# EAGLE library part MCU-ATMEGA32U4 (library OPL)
8-bit Microcontroller with 16/32K Bytes of ISP Flash and USB Controller
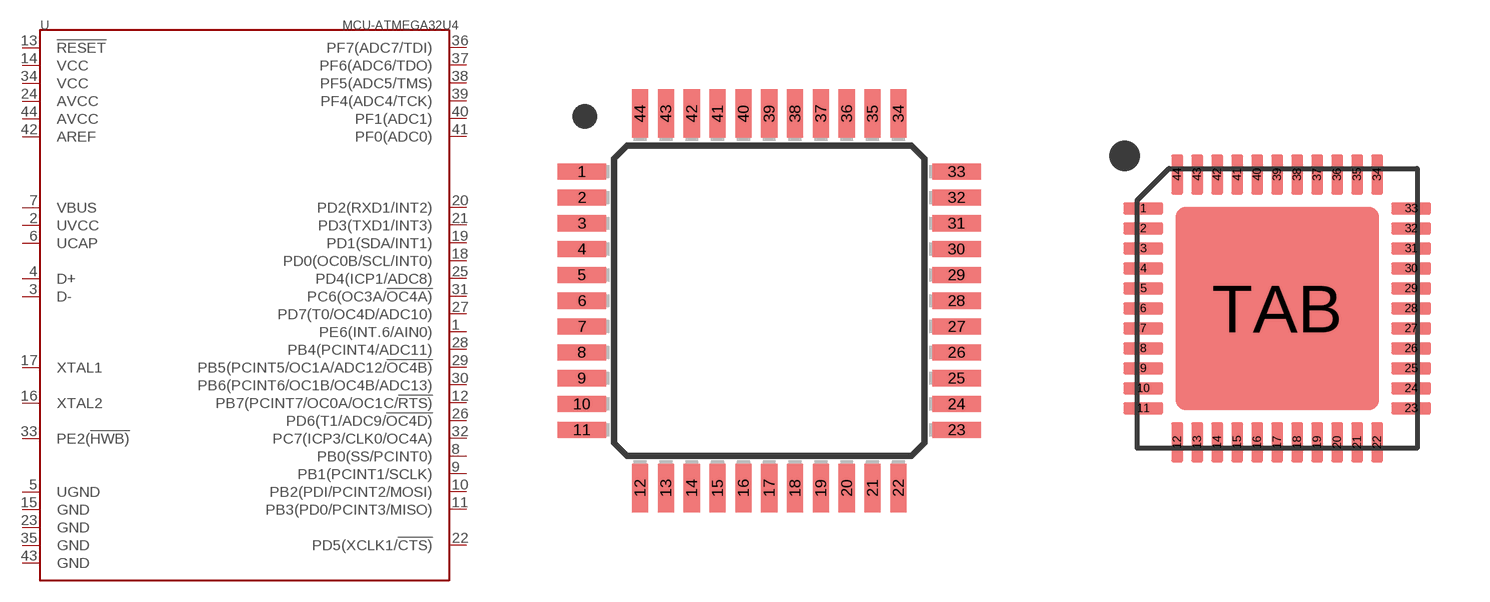
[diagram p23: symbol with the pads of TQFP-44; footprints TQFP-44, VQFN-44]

Designator prefix U

## MCU-ATMEGA32U4-310010010  [TQFP-44]
1  PE6(INT.6/AIN0)
2  UVCC
3  D-
4  D+
5  UGND
6  UCAP
7  VBUS
8  PB0(SS/PCINT0)
9  PB1(PCINT1/SCLK)
10  PB2(PDI/PCINT2/MOSI)
11  PB3(PD0/PCINT3/MISO)
12  PB7(PCINT7/OC0A/OC1C/!RTS)
13  !RESET
14  VCC
15  GND
16  XTAL2
17  XTAL1
18  PD0(OC0B/SCL/INT0)
19  PD1(SDA/INT1)
20  PD2(RXD1/INT2)
21  PD3(TXD1/INT3)
22  PD5(XCLK1/!CTS)
23  GND
24  AVCC
25  PD4(ICP1/ADC8)
26  PD6(T1/ADC9/!OC4D)
27  PD7(T0/OC4D/ADC10)
28  PB4(PCINT4/ADC11)
29  PB5(PCINT5/OC1A/ADC12/!OC4B)
30  PB6(PCINT6/OC1B/OC4B/ADC13)
31  PC6(OC3A/!OC4A)
32  PC7(ICP3/CLK0/OC4A)
33  PE2(!HWB)
34  VCC
35  GND
36  PF7(ADC7/TDI)
37  PF6(ADC6/TDO)
38  PF5(ADC5/TMS)
39  PF4(ADC4/TCK)
40  PF1(ADC1)
41  PF0(ADC0)
42  AREF
43  GND
44  AVCC

## MCU-ATMEGA32U4-310010016  [VQFN-44]
1  PE6(INT.6/AIN0)
2  UVCC
3  D-
4  D+
5  UGND
6  UCAP
7  VBUS
8  PB0(SS/PCINT0)
9  PB1(PCINT1/SCLK)
10  PB2(PDI/PCINT2/MOSI)
11  PB3(PD0/PCINT3/MISO)
12  PB7(PCINT7/OC0A/OC1C/!RTS)
13  !RESET
14  VCC
15  GND
16  XTAL2
17  XTAL1
18  PD0(OC0B/SCL/INT0)
19  PD1(SDA/INT1)
20  PD2(RXD1/INT2)
21  PD3(TXD1/INT3)
22  PD5(XCLK1/!CTS)
23  GND
24  AVCC
25  PD4(ICP1/ADC8)
26  PD6(T1/ADC9/!OC4D)
27  PD7(T0/OC4D/ADC10)
28  PB4(PCINT4/ADC11)
29  PB5(PCINT5/OC1A/ADC12/!OC4B)
30  PB6(PCINT6/OC1B/OC4B/ADC13)
31  PC6(OC3A/!OC4A)
32  PC7(ICP3/CLK0/OC4A)
33  PE2(!HWB)
34  VCC
35  GND
36  PF7(ADC7/TDI)
37  PF6(ADC6/TDO)
38  PF5(ADC5/TMS)
39  PF4(ADC4/TCK)
40  PF1(ADC1)
41  PF0(ADC0)
42  AREF
43  GND
44  AVCC
TAB  GND

## Footprint TQFP-44 (pad centres in mm)
Thin Plasic Quad Flat Package
smd 1.5 x 0.5: 1 -5.8,4; 2 -5.8,3.2; 3 -5.8,2.4; 4 -5.8,1.6; 5 -5.8,0.8; 6 -5.8,0; 7 -5.8,-0.8; 8 -5.8,-1.6; 9 -5.8,-2.4; 10 -5.8,-3.2; 11 -5.8,-4; 23 5.8,-4; 24 5.8,-3.2; 25 5.8,-2.4; 26 5.8,-1.6; 27 5.8,-0.8; 28 5.8,0; 29 5.8,0.8; 30 5.8,1.6; 31 5.8,2.4; 32 5.8,3.2; 33 5.8,4
smd 0.5 x 1.5: 12 -4,-5.8; 13 -3.2,-5.8; 14 -2.4,-5.8; 15 -1.6,-5.8; 16 -0.8,-5.8; 17 0,-5.8; 18 0.8,-5.8; 19 1.6,-5.8; 20 2.4,-5.8; 21 3.2,-5.8; 22 4,-5.8; 34 4,5.8; 35 3.2,5.8; 36 2.4,5.8; 37 1.6,5.8; 38 0.8,5.8; 39 0,5.8; 40 -0.8,5.8; 41 -1.6,5.8; 42 -2.4,5.8; 43 -3.2,5.8; 44 -4,5.8

## Footprint VQFN-44 (pad centres in mm)
smd 1 x 0.3: 1 -3.35,2.5; 2 -3.35,2; 3 -3.35,1.5; 4 -3.35,1; 5 -3.35,0.5; 6 -3.35,0; 7 -3.35,-0.5; 8 -3.35,-1; 9 -3.35,-1.5; 10 -3.35,-2; 11 -3.35,-2.5; 23 3.35,-2.5; 24 3.35,-2; 25 3.35,-1.5; 26 3.35,-1; 27 3.35,-0.5; 28 3.35,0; 29 3.35,0.5; 30 3.35,1; 31 3.35,1.5; 32 3.35,2; 33 3.35,2.5
smd 0.3 x 1: 12 -2.5,-3.35; 13 -2,-3.35; 14 -1.5,-3.35; 15 -1,-3.35; 16 -0.5,-3.35; 17 0,-3.35; 18 0.5,-3.35; 19 1,-3.35; 20 1.5,-3.35; 21 2,-3.35; 22 2.5,-3.35; 34 2.5,3.35; 35 2,3.35; 36 1.5,3.35; 37 1,3.35; 38 0.5,3.35; 39 0,3.35; 40 -0.5,3.35; 41 -1,3.35; 42 -1.5,3.35; 43 -2,3.35; 44 -2.5,3.35
smd 5.08 x 5.08: TAB 0,0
